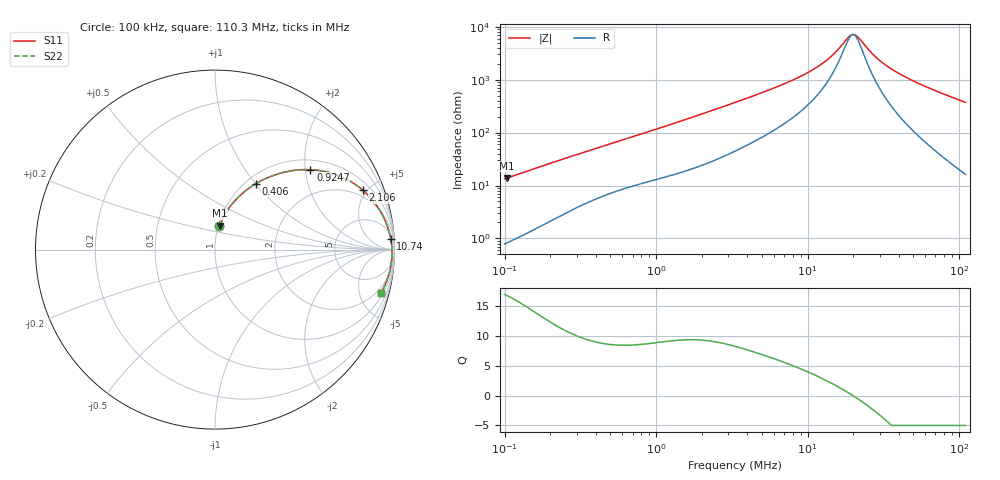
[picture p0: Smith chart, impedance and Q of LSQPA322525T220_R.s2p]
! LSQPA322525T220_R  S-PARAMETER MODEL  ( General Type )
! Model Generated by TAIYO YUDEN Corporation (http://www.ty-top.com)
! Version 2.0
! TAIYO YUDEN Control No. 100810NF25SB-FAC
! Copyright(c) 2007 TAIYO YUDEN CO.,LTD. All Rights Reserved.
! Product Description (link to TY-COMPAS)
! https://ds.yuden.co.jp/TYCOMPAS/or/detail?pn=LSQPA322525T220KR&u=M
! Products Name : Inductors
! Characteristics :
!  Inductance : 22 uH , SRF(min) : 17 MHz , DC Resistance(max) : 0.351 Ohm
!  Rated Current : Saturation :620 mA , Temp Rise : 780 mA (40 degC)
!  Case Size : 3.2 x 2.5 / 0.126 x 0.098 [mm/inch] , Thickness : 2.5 / 0.098 [mm/inch]
!  (Conditions: Temperature = 25 degC , DC Bias Current/Voltage = 0A / 0V)
! External Node Assignments :
!  1  o---GGG---o  2
! GND o---------o GND
! Frequency Range : 0.1MHz  -  110.285862MHz  [ 402 STEP ]
# MHz S RI R 50
! Freq[MHz].  S11 Real  S11 Imag  S21 Real  S21 Imag  S12 Real  S12 Imag  S22 Real  S22 Imag
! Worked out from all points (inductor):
!   401 points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, 100 kHz to 110.3 MHz, reference 50 ohm
!   read as one part in series: L = 21.1 uH near 103.6 kHz
!   highest Q = 16.8 at 103.6 kHz (marker M1), where L = 21.2 uH
!   self-resonance near 19.95 MHz
!   S11 on the Smith chart (normalised r, x): 100 kHz: 1.02, +0.27; 406 kHz: 1.11, +1.01; 924.7 kHz: 1.24, +2.13; 2.106 MHz: 1.51, +4.69; 10.74 MHz: 9, +29; 110.3 MHz: 1.32, -7.45
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0.1  0.0249 0.1291  0.9751 -0.1291  0.9751 -0.1291  0.0249 0.1291
0.103565  0.0264 0.1334  0.9736 -0.1334  0.9736 -0.1334  0.0264 0.1334
0.191176  0.0753 0.2273  0.9247 -0.2273  0.9247 -0.2273  0.0753 0.2273
0.323312  0.1692 0.3269  0.8308 -0.3269  0.8308 -0.3269  0.1692 0.3269
0.405979  0.2293 0.3682  0.7707 -0.3682  0.7707 -0.3682  0.2293 0.3682
0.640129  0.3835 0.4307  0.6165 -0.4307  0.6165 -0.4307  0.3835 0.4307
0.924698  0.5321 0.4452  0.4679 -0.4452  0.4679 -0.4452  0.5321 0.4452
1.045308  0.5828 0.4403  0.4172 -0.4403  0.4172 -0.4403  0.5828 0.4403
2.106183  0.8228 0.3316  0.1772 -0.3316  0.1772 -0.3316  0.8228 0.3316
3.320932  0.9077 0.2352  0.0923 -0.2352  0.0923 -0.2352  0.9077 0.2352
6.691322  0.9644 0.118  0.0356 -0.118  0.0356 -0.118  0.9644 0.118
10.73698  0.9791 0.0612  0.0209 -0.0612  0.0209 -0.0612  0.9791 0.0612
13.72051  0.9831 0.0361  0.0169 -0.0361  0.0169 -0.0361  0.9831 0.0361
15.51009  0.9845 0.0241  0.0155 -0.0241  0.0155 -0.0241  0.9845 0.0241
18.80544  0.9859 0.00566  0.0141 -0.00566  0.0141 -0.00566  0.9859 0.00566
20.17013  0.9862 -0.00104  0.0138 0.00104  0.0138 0.00104  0.9862 -0.00104
21.63386  0.9864 -0.00776  0.0136 0.00776  0.0136 0.00776  0.9864 -0.00776
28.1338  0.9861 -0.0338  0.0139 0.0338  0.0139 0.0338  0.9861 -0.0338
34.71395  0.9845 -0.0563  0.0155 0.0563  0.0155 0.0563  0.9845 -0.0563
42.83311  0.9813 -0.0813  0.0187 0.0813  0.0187 0.0813  0.9813 -0.0813
55.70243  0.9742 -0.1171  0.0258 0.1171  0.0258 0.1171  0.9742 -0.1171
110.2859  0.9237 -0.2445  0.0763 0.2445  0.0763 0.2445  0.9237 -0.2445
